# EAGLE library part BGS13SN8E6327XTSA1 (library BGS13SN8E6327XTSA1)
INFINEON - BGS13SN8E6327XTSA1 - RF SWITCH, SP3T, 0.1-6GHZ, TSNP-8 Source: Datasheet
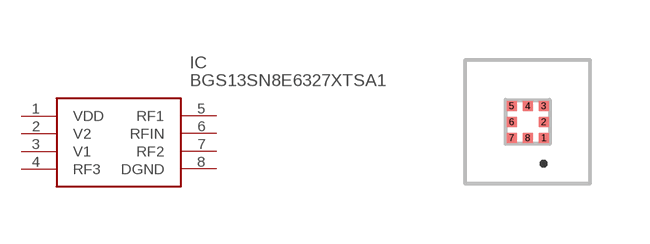
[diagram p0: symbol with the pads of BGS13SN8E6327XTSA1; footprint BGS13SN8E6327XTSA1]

Designator prefix IC

## BGS13SN8E6327XTSA1 (Description: INFINEON - BGS13SN8E6327XTSA1 - RF SWITCH, SP3T, 0.1-6GHZ, TSNP-8; Height: 0.4mm; Manufacturer_Name: Infineon; Manufacturer_Part_Number: BGS13SN8E6327XTSA1; Mouser_Part_Number: 726-BGS13SN8E6327XTS; Mouser_Price-Stock: https://www.mouser.co.uk/ProductDetail/Infineon-Technologies/BGS13SN8E6327XTSA1?qs=0DP5yvOrqYmFtfP%252BZ8kQgQ%3D%3D)  [BGS13SN8E6327XTSA1]
1  VDD
2  V2
3  V1
4  RF3
5  RF1
6  RFIN
7  RF2
8  DGND

## Footprint BGS13SN8E6327XTSA1 (pad centres in mm)
TSNP-8-1
smd 0.25 x 0.25: 1 0.4,-0.4; 2 0.4,0; 3 0.4,0.4; 4 0,0.4; 5 -0.4,0.4; 6 -0.4,0; 7 -0.4,-0.4; 8 0,-0.4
